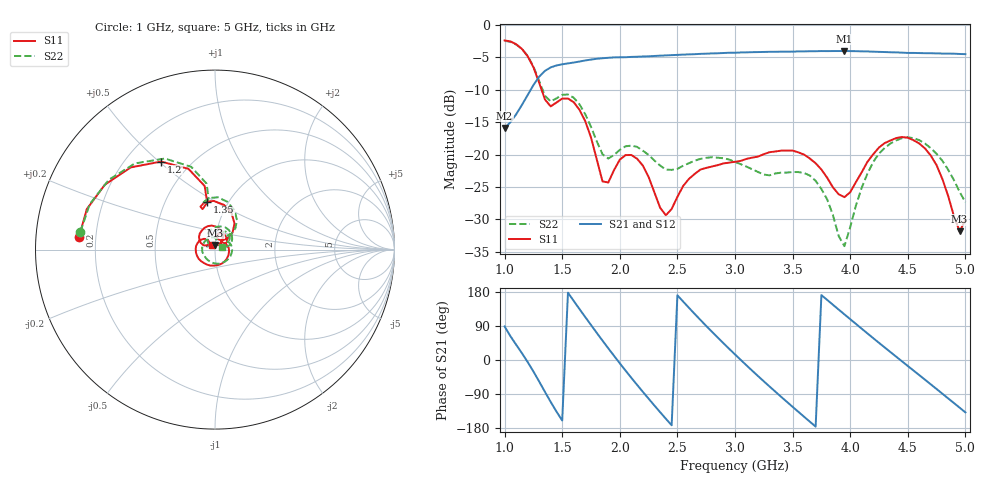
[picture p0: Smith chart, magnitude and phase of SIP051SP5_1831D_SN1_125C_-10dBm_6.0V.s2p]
# GHz  S  dB  R  50
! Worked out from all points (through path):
!   81 points, 1 GHz to 5 GHz, reference 50 ohm
!   highest |S21| = -4.00 dB at 3.95 GHz (marker M1); lowest = -15.9 dB at 1 GHz (marker M2)
!   lowest |S11| = -31.8 dB at 4.95 GHz (marker M3), VSWR 1.05, Z = 50.1 + j2.56 ohm
!   |S11| at or under -10 dB: 1.321 GHz to end of sweep
!   |S22| runs from -34.1 to -2.4 dB; largest |S21 - S12| = 0.0025
!   S11 on the Smith chart (normalised r, x): 1 GHz: 0.14, +0.05; 1.2 GHz: 0.35, +0.51; 1.35 GHz: 0.80, +0.45; 5 GHz: 0.97, +0.05
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1  -2.37 174.7  -15.89 88.6  -15.90 88.6  -2.42 172.5
1.2  -4.80 121.5  -10.80 -5.3  -10.79 -5.4  -4.75 118.8
1.35  -11.48 99.4  -7.07 -84.0  -7.05 -84.0  -10.90 97.1
1.55  -11.33 91.5  -5.91 177.7  -5.91 177.7  -10.70 86.9
1.7  -14.82 53.1  -5.46 113.4  -5.47 113.3  -13.76 53.3
1.85  -24.14 53.9  -5.11 51.1  -5.10 51.0  -19.93 49.7
2  -20.78 78.3  -4.96 -8.7  -4.96 -8.7  -19.26 65.2
2.2  -21.68 34.7  -4.84 -84.0  -4.85 -83.9  -19.39 40.5
2.35  -28.20 25.5  -4.71 -137.6  -4.71 -137.6  -21.68 32.3
2.5  -26.52 50.2  -4.60 170.8  -4.59 170.8  -22.20 33.4
2.7  -22.30 7.3  -4.44 105.7  -4.44 105.7  -20.65 17.0
2.85  -21.61 -37.9  -4.35 59.3  -4.34 59.2  -20.47 -10.3
3  -21.10 -79.7  -4.26 14.7  -4.25 14.7  -21.13 -46.4
3.15  -20.45 -117.8  -4.18 -28.4  -4.18 -28.3  -22.26 -92.7
3.35  -19.51 -160.7  -4.12 -83.5  -4.11 -83.6  -22.90 -169.9
3.7  -21.32 135.8  -4.03 -175.8  -4.02 -175.7  -24.04 87.9
3.95  -26.56 141.9  -4.00 120.4  -3.99 120.4  -34.13 104.7
4.15  -21.09 154.4  -4.06 70.1  -4.07 70.1  -22.91 127.5
4.35  -17.80 125.1  -4.19 20.8  -4.20 20.8  -18.27 93.1
4.7  -20.15 64.2  -4.34 -64.4  -4.34 -64.4  -19.00 31.5
4.95  -31.85 86.6  -4.46 -125.9  -4.46 -125.9  -25.74 16.8
5  -30.06 118.7  -4.48 -138.2  -4.49 -138.3  -27.35 23.1
